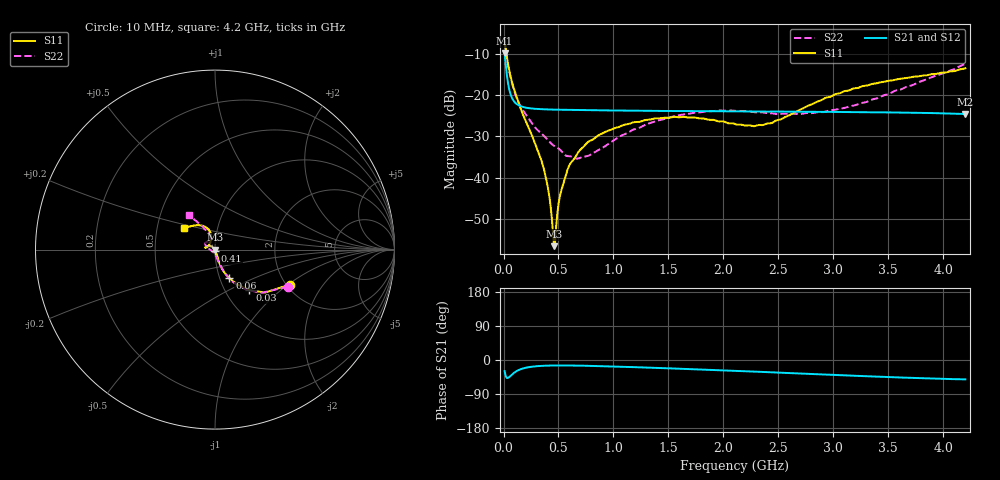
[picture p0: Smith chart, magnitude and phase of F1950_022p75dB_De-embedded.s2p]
! Integrated Device Technology
! Corporate Headquarters
! 6024 Silver Creek Valley Road
! San Jose, CA 95138  USA
! Phone:  1-408-284-8200
! Toll Free:  1-800-223-1366
! Webpage:  http://www.idt.com/
! Timing and RF Division
! 515 Groton Road, Suite 102
! Westford, MA 01886-6024
! Device:  F1950
! Description: 7-bit 0.25 dB Digital Step Attenuator
! Frequency:  150.0 -  4000.00 MHz
! Package:  4x4 mm Thin QFN Plastic Package: 24 pin
! Ports:  2 RF, 12 DC
!  Pin  1  = D0
!  Pin  2  = VDD
!  Pin  3  = Vmode
!  Pin  4  = GND
!  Pin  5  = RF1  =  Port 1
!  Pin  6  = GND
!  Pin  7  = GND
!  Pin  8  = GND
!  Pin  9  = GND
!  Pin 10  = GND
!  Pin 11  = GND
!  Pin 12  = GND
!  Pin 13  = GND
!  Pin 14  = RF2  =  Port 2
!  Pin 15  = GND
!  Pin 16  = LE
!  Pin 17  = CLK
!  Pin 18  = DATE
!  Pin 19  = D6
!  Pin 20  = D5
!  Pin 21  = D4
!  Pin 22  = D3
!  Pin 23  = D2
!  Pin 24  = D1
! State:  91
! Atten State:  22.75 dB
! Voltage:  +5.00 Volts
! Current:  Not Measured mA
! Data:  The device was measured on a the F195X evaluation board which has
!  individual transmission lines to the RF pins.  Data was collected
!  using a calibrated network analyzer.  The evaluation board was
!  de-embedded using a TRL calibration technique.
!  The reference plane is the edge of the package pin.
! Misc:  Board 2019
!  Action Tracker AT0250
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# GHz S dB R 50
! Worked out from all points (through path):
!   420 points, 10 MHz to 4.2 GHz, reference 50 ohm
!   highest |S21| = -9.85 dB at 10 MHz (marker M1); lowest = -24.6 dB at 4.2 GHz (marker M2)
!   group delay of S21, straight-line fit = 24.3 ps
!   lowest |S11| = -56.7 dB at 460 MHz (marker M3), VSWR 1.00, Z = 49.9 - j0.0895 ohm
!   |S11| at or under -10 dB: 26.97 MHz to end of sweep
!   |S22| runs from -35.4 to -6.8 dB; largest |S21 - S12| = 0.00012
!   S11 on the Smith chart (normalised r, x): 10 MHz: 2.09, -1.04; 30 MHz: 1.30, -0.64; 60 MHz: 1.11, -0.36; 410 MHz: 1.00, -0.01; 4.2 GHz: 0.68, +0.17
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0.01  -6.71 -24.9  -9.85 -29.4  -9.85 -29.4  -6.85 -27.1
0.03  -10.57 -49.7  -15.02 -47.3  -15.02 -47.3  -10.92 -51.9
0.06  -14.99 -63.1  -19.43 -42.9  -19.43 -42.9  -15.20 -64.5
0.1  -18.86 -70.0  -21.64 -32.8  -21.64 -32.8  -19.24 -69.7
0.16  -23.53 -71.9  -22.72 -23.9  -22.72 -23.9  -22.92 -74.6
0.34  -35.50 -69.8  -23.39 -15.6  -23.39 -15.6  -29.18 -83.6
0.41  -43.44 -75.5  -23.47 -14.7  -23.47 -14.8  -31.07 -86.5
0.45  -53.54 -105.3  -23.50 -14.5  -23.50 -14.5  -32.12 -92.2
0.46  -56.65 -142.4  -23.51 -14.4  -23.50 -14.5  -32.31 -93.9
0.48  -51.54 153.4  -23.52 -14.4  -23.52 -14.4  -32.61 -96.9
0.52  -43.68 139.7  -23.54 -14.3  -23.54 -14.3  -33.40 -100.4
0.57  -39.13 134.7  -23.56 -14.4  -23.56 -14.4  -34.70 -110.3
0.61  -36.49 136.5  -23.58 -14.5  -23.58 -14.5  -34.84 -119.0
0.71  -32.96 137.9  -23.61 -15.0  -23.62 -15.0  -35.09 -139.0
1  -28.11 148.0  -23.71 -17.2  -23.71 -17.2  -31.01 179.2
1.41  -25.61 163.2  -23.81 -21.1  -23.81 -21.1  -26.08 160.7
1.73  -25.40 168.6  -23.86 -24.4  -23.86 -24.4  -24.26 152.4
2.11  -27.05 158.3  -23.93 -28.9  -23.93 -28.9  -23.82 142.6
2.43  -26.81 126.7  -23.97 -32.4  -23.97 -32.4  -24.37 131.9
2.81  -22.13 105.5  -24.02 -37.0  -24.02 -37.0  -24.33 116.5
3.51  -16.47 117.6  -24.18 -45.1  -24.17 -45.1  -19.64 113.3
4.2  -13.47 145.8  -24.57 -51.0  -24.57 -51.1  -12.40 127.0
